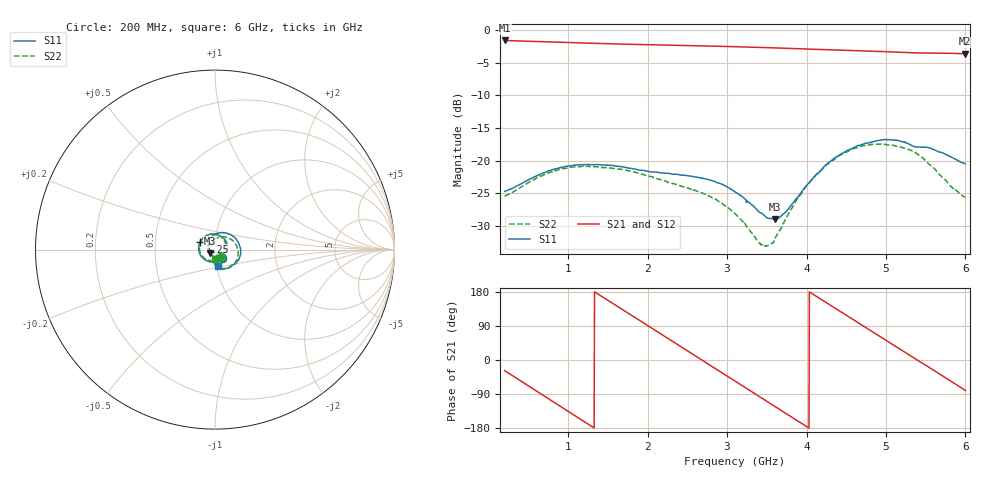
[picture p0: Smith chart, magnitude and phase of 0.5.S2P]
!Agilent Technologies,E5071C,MY46316741,A.11.02
!Date: Fri Apr 15 16:19:09 2022
!Data & Calibration Information:
!Freq	S11:SOLT2(ON)	S21:SOLT2(ON)	S12:SOLT2(ON)	S22:SOLT2(ON)
!PortZ  Port1:50+j0  Port2:50+j0
!Above PortZ is port z conversion or system Z0 setting when saving the data.
!When reading, reference impedance value at option line is always used.
# Hz S dB R 50
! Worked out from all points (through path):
!   1200 points, 200 MHz to 6 GHz, reference 50 ohm
!   highest |S21| = -1.62 dB at 200 MHz (marker M1); lowest = -3.7 dB at 5.99 GHz (marker M2)
!   group delay of S21, straight-line fit = 370 ps
!   lowest |S11| = -29.0 dB at 3.606 GHz (marker M3), VSWR 1.07, Z = 47.2 - j1.95 ohm
!   |S11| at or under -10 dB: start of sweep to end of sweep
!   |S22| runs from -33.1 to -17.5 dB; largest |S21 - S12| = 0.0025
!   S11 on the Smith chart (normalised r, x): 200 MHz: 1.07, -0.10; 1.25 GHz: 0.85, +0.08; 6 GHz: 1.01, -0.19
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2e8  -24.70 -49.9  -1.62 -28.0  -1.62 -27.9  -25.43 -53.9
4.563803e8  -23.22 -98.5  -1.72 -62.6  -1.72 -62.6  -23.67 -105.7
6.740617e8  -21.97 -133.8  -1.81 -92.0  -1.81 -92.0  -22.30 -142.9
9.014178e8  -21.08 -166.0  -1.89 -122.5  -1.89 -122.5  -21.34 -176.9
1.167473e9  -20.64 160.6  -1.99 -158.2  -1.99 -158.1  -20.90 147.8
1.249708e9  -20.59 151.2  -2.02 -169.2  -2.02 -169.1  -20.89 137.7
1.486739e9  -20.70 125.8  -2.11 159.2  -2.11 159.3  -21.08 110.4
1.747957e9  -21.11 100.5  -2.20 124.5  -2.20 124.6  -21.52 82.3
2.134946e9  -21.80 68.2  -2.30 73.1  -2.30 73.1  -22.84 45.0
2.401001e9  -22.17 45.1  -2.36 37.6  -2.36 37.6  -23.85 22.0
2.628357e9  -22.55 23.7  -2.43 7.3  -2.43 7.3  -24.71 1.8
2.855713e9  -23.27 -1.0  -2.49 -23.1  -2.50 -23.0  -25.90 -21.9
3.102419e9  -24.79 -33.5  -2.57 -55.9  -2.57 -55.9  -28.13 -54.3
3.353962e9  -27.23 -77.5  -2.66 -89.5  -2.66 -89.4  -31.78 -105.9
3.605505e9  -28.99 -144.4  -2.75 -123.0  -2.75 -122.9  -31.86 166.4
3.847373e9  -26.19 149.2  -2.86 -155.2  -2.86 -155.1  -26.60 108.0
4.069892e9  -22.86 106.0  -2.96 175.2  -2.96 175.3  -22.88 73.1
4.577815e9  -18.12 37.3  -3.15 107.9  -3.15 108.0  -18.22 10.0
5.037364e9  -16.79 -13.3  -3.35 47.1  -3.35 47.2  -17.60 -40.3
5.492077e9  -17.95 -51.0  -3.54 -12.7  -3.54 -12.6  -19.92 -82.3
5.990325e9  -20.44 -80.8  -3.65 -78.9  -3.66 -78.9  -25.55 -88.5
6e9  -20.49 -81.0  -3.65 -80.2  -3.66 -80.1  -25.61 -88.0
